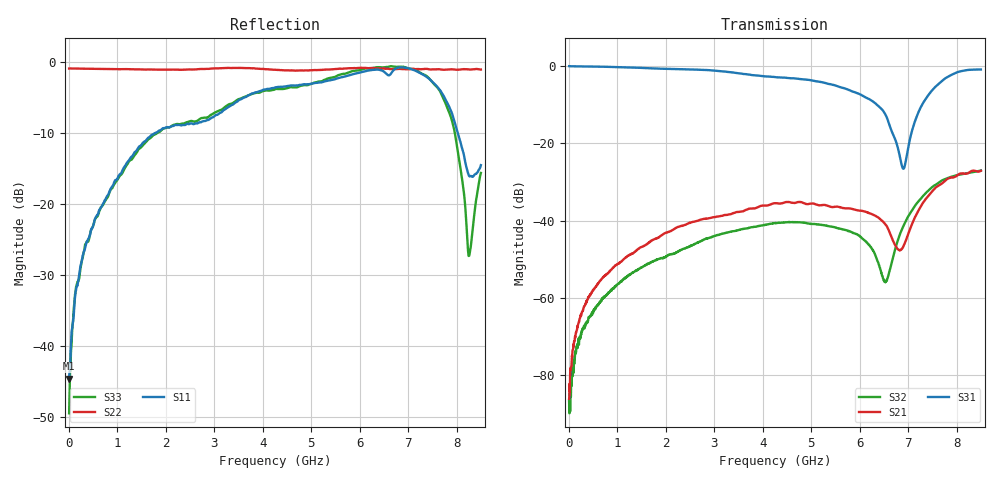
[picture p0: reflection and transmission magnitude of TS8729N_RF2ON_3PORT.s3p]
!Created with skrf (http://scikit-rf.org).
# GHz S RI R 50.0
!freq ReS11 ImS11 ReS12 ImS12 ReS13 ImS13
! ReS21 ImS21 ReS22 ImS22 ReS23 ImS23
! ReS31 ImS31 ReS32 ImS32 ReS33 ImS33
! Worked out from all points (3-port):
!   1601 points, 10 MHz to 8.5 GHz, reference 50 ohm
!   strongest paths, dB at 10 MHz, 2.132 GHz, 4.255 GHz, 6.378 GHz, 8.5 GHz:
!     S31: -0.1, -0.8, -2.9, -10.3, -0.9
!     S21: -86.1, -42.5, -35.5, -39.2, -27.1
!     S32: -86.8, -48.7, -40.7, -50.7, -27.1
!   lowest |S11| = -44.6 dB at 10 MHz (marker M1), VSWR 1.01, Z = 50.6 - j0.129 ohm
!   |S11| at or under -10 dB: start of sweep to 1.783 GHz; 8.025 GHz to end of sweep
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0.01  0.00573 -0.00128  5.53e-06 4.57e-05  0.9916 -0.00547
      1.33e-05 4.74e-05  -0.9016 0.00546  3.07e-05 -1.2e-06
      0.9917 -0.00557  4.46e-05 1.12e-05  0.00319 -0.000981
0.328375  -0.00606 -0.0467  -4.4e-05 0.0008  0.975 -0.121
          -7.42e-05 0.000785  -0.8936 0.1031  -0.000201 -0.000398
          0.975 -0.1216  -0.000171 -0.000381  -0.00801 -0.0486
1.214519  -0.0805 -0.1803  -0.000699 0.00339  0.8621 -0.4184
          -0.000696 0.0034  -0.8317 0.3247  -0.00189 -0.000305
          0.8622 -0.4185  -0.00186 -0.000303  -0.0943 -0.1667
4.255  -0.6573 -0.0829  0.00667 0.0154  0.0375 -0.7157
       0.00672 0.0154  -0.3093 0.8285  0.000626 0.00927
       0.0356 -0.7158  0.0006 0.00922  -0.6425 0.0376
5.953  -0.6816 0.4852  0.0113 0.00745  -0.282 -0.3417
       0.0114 0.00745  0.1305 0.8988  0.00507 0.00423
       -0.2823 -0.3418  0.00508 0.00419  -0.5813 0.6533
6.526075  -0.4973 0.6805  0.00808 0.00397  -0.2012 -0.1274
          0.00809 0.00394  0.2766 0.8547  4.25e-05 0.0016
          -0.2013 -0.1273  4.46e-05 0.0016  -0.3833 0.837
6.902819  -0.3467 0.8501  -0.00035 0.00462  0.00727 -0.046
          -0.000363 0.00465  0.4567 0.769  -0.00743 0.00427
          0.00721 -0.0462  -0.00739 0.00421  -0.0793 0.9249
7.86325  0.274 0.3816  0.00319 0.0356  0.3132 -0.6817
         0.00316 0.0355  0.5829 0.6703  0.00466 0.036
         0.3123 -0.6826  0.00466 0.036  0.4002 0.1484
8.261219  0.0145 0.1563  0.0177 0.038  -0.029 -0.889
          0.0177 0.0379  0.6026 0.6522  0.0229 0.0346
          -0.0298 -0.8893  0.0229 0.0347  -0.00497 0.043
8.5  -0.1212 0.1434  0.0248 0.0365  -0.2099 -0.8734
     0.0248 0.0364  0.6528 0.5999  0.0313 0.0315
     -0.211 -0.8732  0.0313 0.0315  -0.1309 0.1011
